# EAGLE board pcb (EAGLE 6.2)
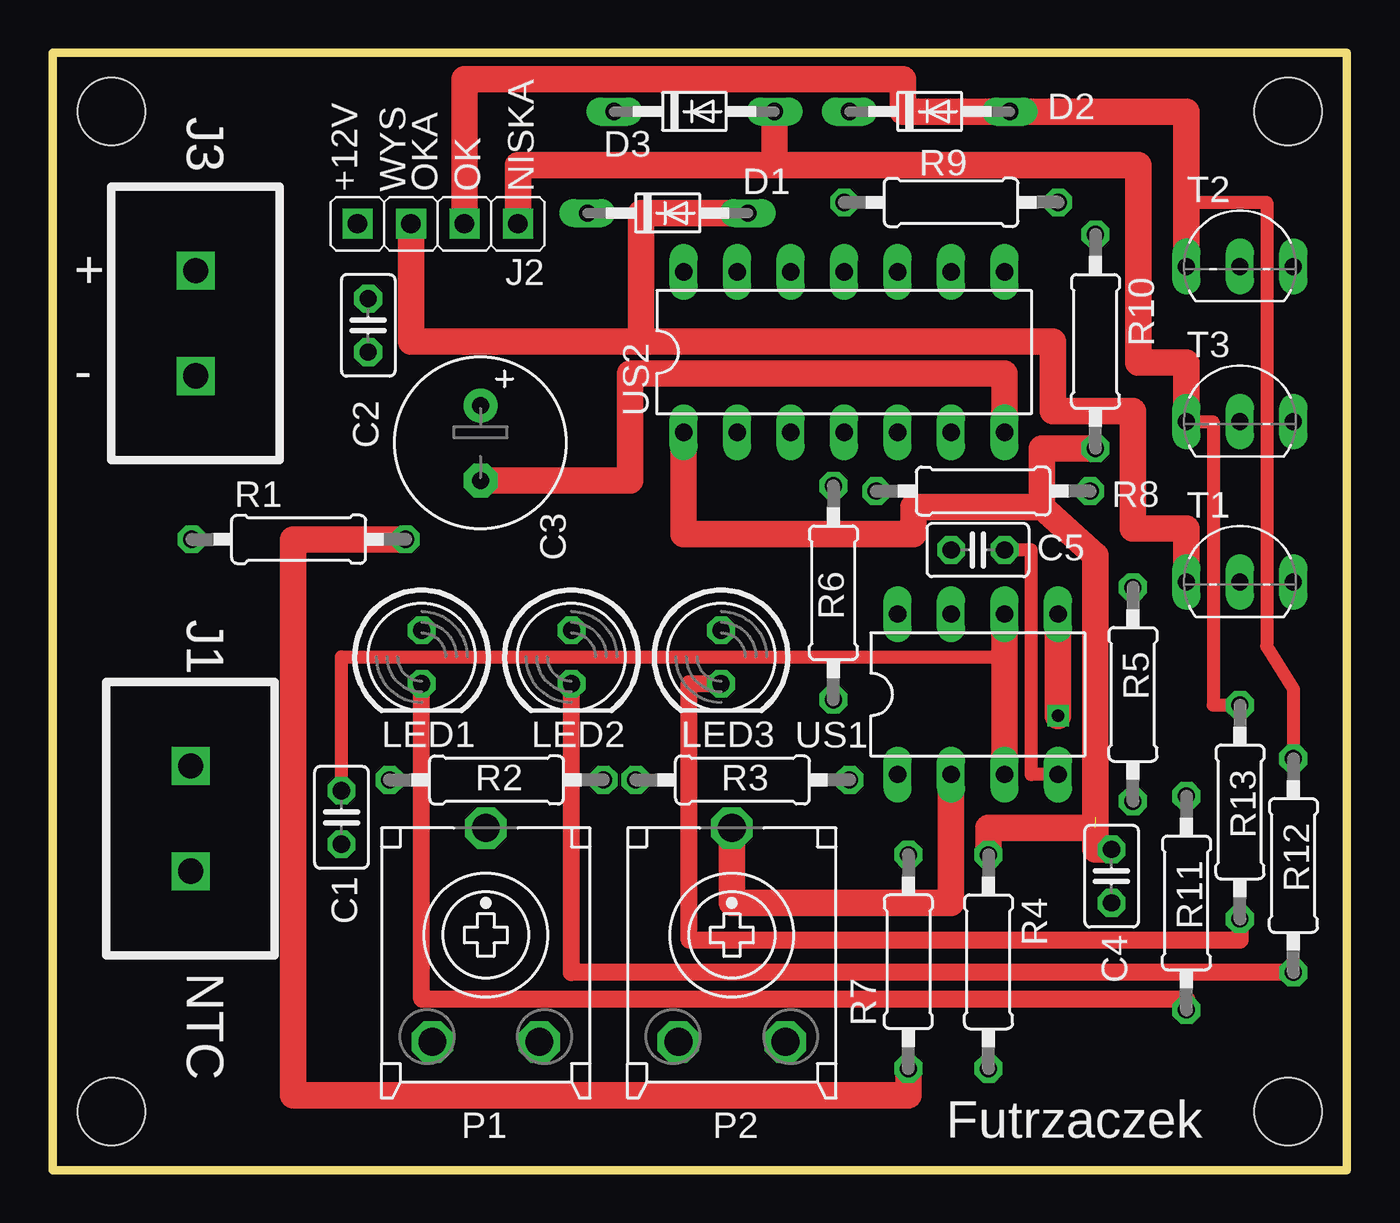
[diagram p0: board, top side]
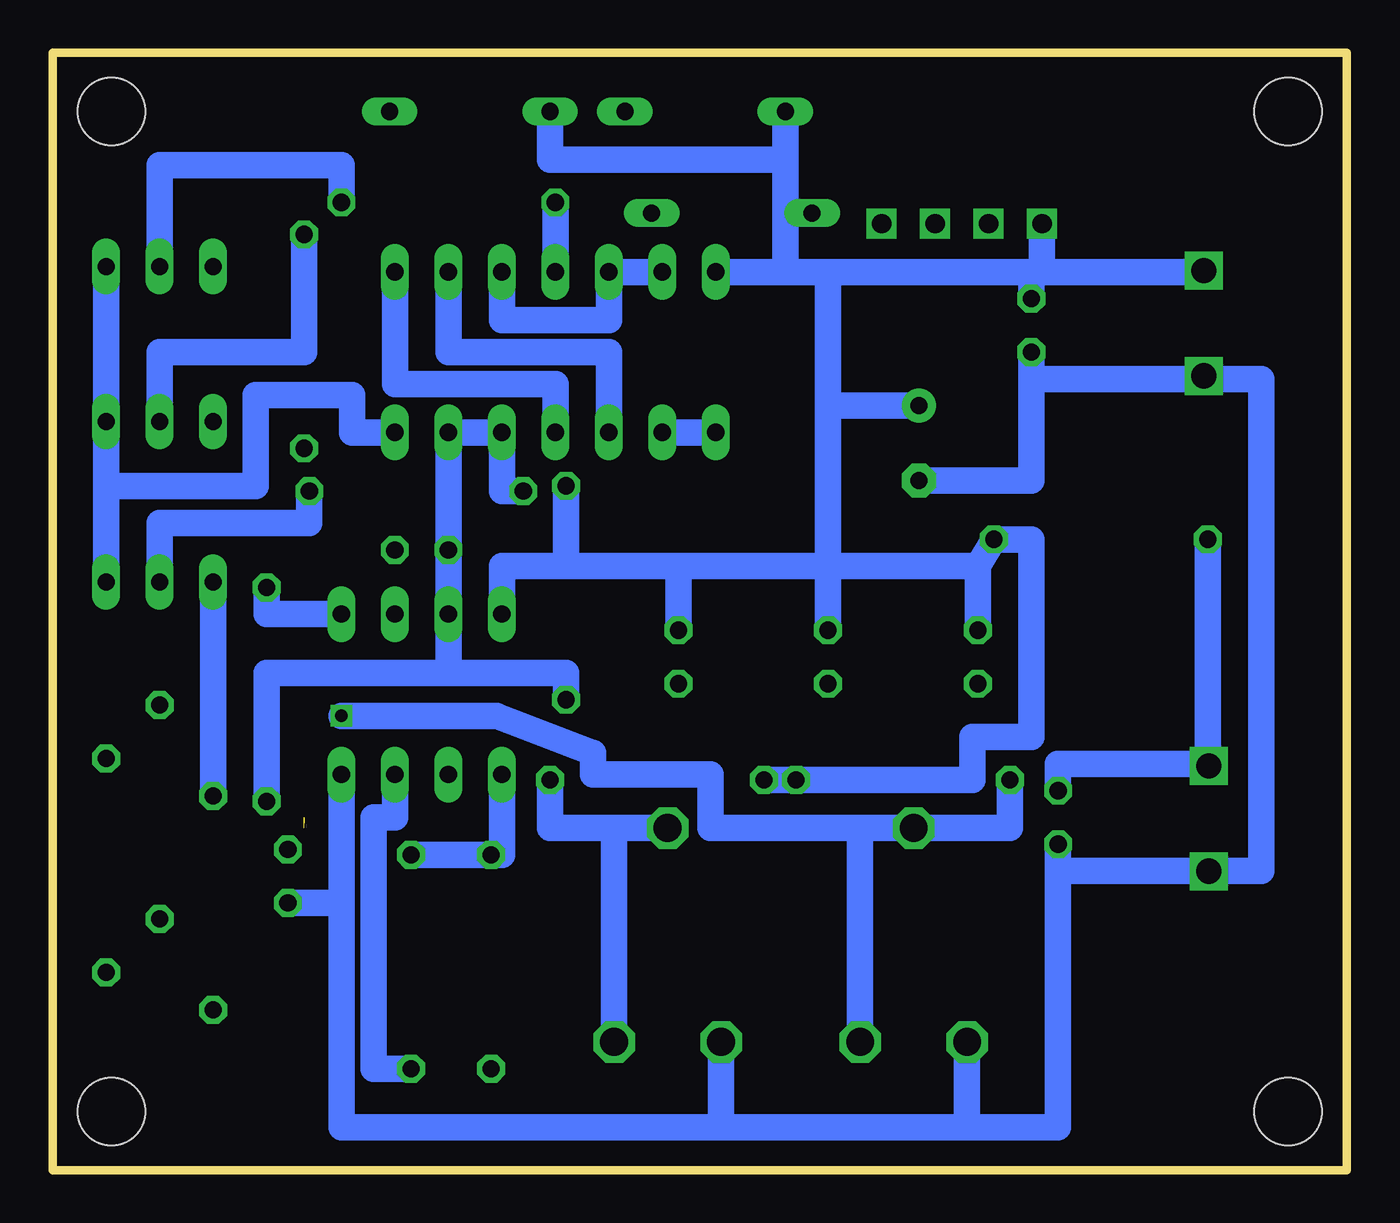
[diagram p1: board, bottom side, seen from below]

Size 61.47 x 53.09 mm. Coordinates in mm from the lower left corner, seen from the top.
Outline: 0,53.09 61.47,53.09 61.47,0 0,0 0,53.09
Copper layers (1*16): Top 0.035mm / dielectric 1.5mm / Bottom 0.035mm
Design rules: minimum track width 10mil, minimum drill 24mil, track to track 8mil, track to pad 8mil, pad to pad 8mil, via to via 8mil, smd to smd 8mil, copper to edge 40mil, drill to drill 8mil, minimum pad ring 10mil, minimum via ring 8mil, stop-mask expansion 4mil, vias tented up to drill 0mil, thermal gap 10mil
Holes 3.2 mm at 2.79,50.29 2.79,2.79 58.67,2.79 58.67,50.29

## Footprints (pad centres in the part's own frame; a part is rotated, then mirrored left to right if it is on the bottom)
C025-025X050 = drill 0.813 octagon: 1 -1.27,0; 2 1.27,0
E3,5-8 = drill 0.813 pad 1.6: + -1.778,0 | drill 0.813 pad 1.6 octagon: - 1.778,0
DO34-7 = drill 0.813 long: A 3.81,0; C -3.81,0
JP1 = drill 0.914 pad 1.422 square: 1 0,-1.27; 2 0,1.27
LED5MM = drill 0.813 octagon: A -1.27,0; K 1.27,0
ECP10S = drill 1.321 octagon: A -2.54,-5.08; E 2.54,-5.08; S 0,5.08
0207/10 = drill 0.813 octagon: 1 -5.08,0; 2 5.08,0
TO92- = drill 0.813 long: 1 2.54,0; 2 0,0; 3 -2.54,0
DIL08 = drill 0.813 long: 1 -3.81,-3.81; 2 -1.27,-3.81; 3 1.27,-3.81; 4 3.81,-3.81; 5 3.81,3.81; 6 1.27,3.81; 7 -1.27,3.81; 8 -3.81,3.81
DIL14 = drill 0.813 long: 1 -7.62,-3.81; 2 -5.08,-3.81; 3 -2.54,-3.81; 4 0,-3.81; 5 2.54,-3.81; 6 5.08,-3.81; 7 7.62,-3.81; 8 7.62,3.81; 9 5.08,3.81; 10 2.54,3.81; 11 0,3.81; 12 -2.54,3.81; 13 -5.08,3.81; 14 -7.62,3.81

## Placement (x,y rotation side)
C1  [C025-025X050]  13.72,16.76 270 top
C2  [C025-025X050]  14.99,40.13 270 top
C3  [E3,5-8]  20.32,34.54 270 top
C4  [C025-025X050]  50.29,13.97 270 top
C5  [C025-025X050]  43.94,29.46 0 top
D1  [DO34-7]  29.21,45.47 0 top
D2  [DO34-7]  41.66,50.29 0 top
D3  [DO34-7]  30.48,50.29 0 top
E$15  [JP1]  15.75,44.96 90 top
E$22  [JP1]  18.29,44.96 90 top
J2  [JP1]  20.83,44.96 90 top
LED1  [LED5MM]  17.53,24.38 270 top
LED2  [LED5MM]  24.64,24.38 270 top
LED3  [LED5MM]  31.75,24.38 270 top
P1  [ECP10S]  20.57,11.18 0 top
P2  [ECP10S]  32.26,11.18 0 top
R1  [0207/10]  11.68,29.97 0 top
R2  [0207/10]  21.08,18.54 0 top
R3  [0207/10]  32.77,18.54 0 top
R4  [0207/10]  44.45,9.91 270 top
R5  [0207/10]  51.31,22.61 270 top
R6  [0207/10]  37.08,27.43 270 top
R7  [0207/10]  40.64,9.91 90 top
R8  [0207/10]  44.2,32.26 180 top
R9  [0207/10]  42.67,45.97 0 top
R10  [0207/10]  49.53,39.37 270 top
R11  [0207/10]  53.85,12.7 270 top
R12  [0207/10]  58.93,14.48 270 top
R13  [0207/10]  56.39,17.02 270 top
T1  [TO92-]  56.39,27.94 0 top
T2  [TO92-]  56.39,42.93 0 top
T3  [TO92-]  56.39,35.56 0 top
US1  [DIL08]  43.94,22.61 0 top
US2  [DIL14]  37.59,38.86 0 top

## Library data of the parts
C1-C5 R1-R13 = rcl
D1-D3 = diode
E$15 E$22 J2 = hybrid
LED1-LED3 = led
P1 P2 = pot
T1-T3 = transistor-npn
US1 US2 = 40xx

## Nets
S$3: C4.1 R4.1 R7.2 R10.2 US2.1 US2.2
S$4: C5.2 US1.4
S$5: C4.2
S$6: P1.A
S$7: P2.A
S$8: C1.2
S$9: R1.1
S$10: R11.1
S$11: P2.E
S$12: P2.S R3.2
S$13: US2.4 US2.8
S$16: C2.1
S$17: C2.2 C3.-
S$18: C3.+
S$19: D3.A J2.1 R13.1 T3.3
S$20: C1.1
S$21: LED1.A LED2.A LED3.A R1.2 R3.1 R6.1 R7.1
S$22: R9.1
S$23: R9.2
S$24: R4.2 US1.3
S$26: R6.2 US2.5 US2.6
S$27: US2.12 US2.13
S$28: US2.3 US2.9
S$30: R10.1 T3.2
S$31: R8.2
S$32: R8.1
S$33: E$15.2
S$34: LED1.K
S$35: D2.A E$22.1 R12.1
S$36: D1.A E$15.1 T1.3
S$37: T2.1 US2.7
S$38: P1.S R2.1 R5.1 US1.5
S$39: D1.C D2.C D3.C US2.14
S$40: LED2.K
S$41: LED3.K R13.2

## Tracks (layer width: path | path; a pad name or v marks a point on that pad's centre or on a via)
S$1  (via drill 1.2)
  other vias: 6.56,14.21
S$2  (via drill 1.2)
  other vias: 6.56,19.21
S$3  (3 unrouted)
  Top 1.27: R4.1 44.45,16.26 49.53,16.26 | 49.53,16.26 49.53,29.21 46.99,31.5 | R10.2 46.99,34.29 46.99,31.5 | C4.1 49.53,15.24 49.53,16.26 | 46.99,31.5 40.89,31.5 40.89,30.23 29.97,30.23 US2.1
  Bottom 1.27: R4.1 R7.2 40.13,14.99 40.13,19.05 | US2.1 US2.2
S$4
  Top 0.61: US1.4 46.48,18.8 46.48,29.46 C5.2
S$5
  Bottom 1.27: 13.72,2.29 13.72,2.03 47.75,2.03 47.75,12.7 | 47.75,12.7 47.75,19.3 | C4.2 47.75,12.7
S$6
  Bottom 1.27: P1.A 18.03,2.29
S$7
  Bottom 1.27: P2.A 29.72,2.29
S$8
  Bottom 1.27: C1.2 13.72,14.22 | 13.72,14.22 13.72,2.54 | 13.72,14.22 4.06,14.22 4.06,37.59 7.11,37.59
S$9
  Bottom 1.27: 13.72,18.29 13.72,19.3 6.6,19.3 R1.1
S$10
  Bottom 1.27: R11.1 53.85,28.19
S$11
  Bottom 1.27: 34.8,16 P2.E
S$12
  Top 1.27: P2.S 32.26,12.7 42.67,12.7 42.67,19.05
  Bottom 1.27: P2.S 37.85,16.26 R3.2
S$13
  Bottom 1.27: US2.4 37.59,37.34 45.21,37.34 US2.8
S$14  (via drill 1.2)
  other vias: 6.79,37.73
S$15  (via drill 1.2)
  other vias: 6.79,42.73
S$16
  Bottom 1.27: 6.86,42.67 14.99,42.67 | 14.99,42.67 24.64,42.67 24.64,28.96 | C2.1 14.99,42.67
S$17
  Top 1.27: C3.- 27.43,32.77 27.43,37.85 45.21,37.85 45.21,34.54
  Bottom 1.27: C2.2 14.99,37.59 | 14.99,37.59 6.86,37.59 | C3.- 14.99,32.77 14.99,37.59
S$18
  Bottom 1.27: C3.+ 24.38,36.32
S$19
  Top 0.61: T3.3 55.12,35.56 55.12,22.1 R13.1
  Top 1.27: J2.1 22.1,47.75 34.29,47.75 | T3.3 53.85,38.35 51.56,38.35 51.56,47.75 34.29,47.75 | 34.29,47.75 D3.A
S$20
  Top 0.61: C1.1 13.72,24.38 45.21,24.38
  Top 1.27: 45.21,26.67 45.21,24.38 45.21,18.29
S$21
  Top 1.27: R7.1 40.64,3.56 11.43,3.56 11.43,29.97 R1.2
  Bottom 1.27: R3.1 17.78,18.54 17.78,20.57 14.99,20.57 14.99,29.97 R1.2 17.53,28.7 | 40.13,26.16 40.13,28.7 37.08,28.7 | R6.1 37.08,28.7 | 17.53,28.7 24.64,28.7 | 24.64,28.7 31.75,28.7 | 31.75,28.7 37.08,28.7 | LED1.A 17.53,28.7 | LED2.A 24.64,28.7 | LED3.A 31.75,28.7
S$22
  Bottom 1.27: R9.1 37.59,42.42
S$23
  Bottom 1.27: R9.2 47.75,47.75 56.39,47.75 56.39,42.67
S$24
  Bottom 1.27: R4.2 46.23,4.83 46.23,16.76 45.21,16.76 US1.3
S$26
  Bottom 1.27: US2.5 US2.6 42.67,23.62 | R6.2 37.08,23.62 42.67,23.62 | 51.31,17.78 51.31,23.62 42.67,23.62
S$27
  Bottom 1.27: US2.13 US2.12 35.05,40.39 40.13,40.39 40.13,42.93
S$28
  Bottom 1.27: US2.3 35.05,38.86 42.67,38.86 US2.9
S$30
  Bottom 1.27: R10.1 49.53,38.86 56.39,38.86 T3.2
S$31
  Bottom 1.27: R8.2 40.13,32.26 40.13,34.8
S$32
  Bottom 1.27: R8.1 49.28,30.73 56.39,30.73 56.39,27.69
S$33
  Bottom 1.27: E$15.2 14.48,42.93
S$34
  Top 0.813: 53.85,8.13 17.53,8.13 LED1.K
S$35
  Top 0.61: 53.85,45.97 57.66,45.97 57.66,24.89 58.93,22.86 R12.1
  Top 1.27: 53.85,42.42 53.85,45.97 53.85,50.29 D2.A 40.39,50.29 40.39,51.82 19.56,51.82 E$22.1
S$36
  Top 1.27: T1.3 53.85,30.48 51.31,30.48 51.31,36.07 47.5,36.07 47.5,39.37 27.94,39.37 | 27.94,39.37 17.02,39.37 E$15.1 | D1.A 27.94,45.47 27.94,39.37
S$37
  Bottom 1.27: US2.7 47.24,35.05 47.24,36.83 51.82,36.83 51.82,32.51 58.93,32.51 | T2.1 58.93,32.51 | 58.93,32.51 58.93,27.43
S$38  (via drill 0.6)
  Top 1.27: US1.5 v47.75,21.59
  Bottom 1.27: 23.11,16.26 P1.S 16,16.26 R2.1 | 23.11,16.26 23.11,6.35 | 23.11,16.26 30.23,16.26 30.23,18.8 35.81,18.8 35.81,19.81 40.39,21.59 v47.75,21.59 | US1.5 51.31,26.42 R5.1
S$39
  Bottom 1.27: D2.C 37.85,48.01 26.67,48.01 D3.C 26.67,45.47 | US2.14 26.67,42.67 | 26.67,42.67 22.61,42.67 | 26.67,45.47 26.67,42.67 | D1.C 26.67,45.47
S$40
  Top 0.813: 58.93,9.4 24.64,9.4 LED2.K
S$41
  Top 0.813: LED3.K 30.23,23.11 30.23,10.92 56.39,10.92 R13.2

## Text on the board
tNames: J3 | +12V | WYS | OKA | OK | NISKA | + | - | J1 | NTC | Futrzaczek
